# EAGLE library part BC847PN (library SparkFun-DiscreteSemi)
NPN/PNP transistor pair in SOT-363 package
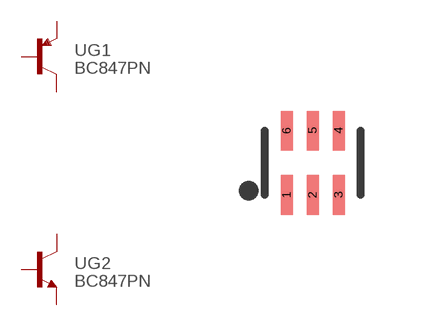
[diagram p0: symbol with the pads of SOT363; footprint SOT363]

Designator prefix -; gates G1=PNP G2=NPN

## BC847PN  [SOT363]
1  G1:E  pas
2  G1:B  pas
3  G2:C  pas
4  G2:E  pas
5  G2:B  pas
6  G1:C  pas

## Footprint SOT363 (pad centres in mm)
smd 0.3 x 0.99: 1 -0.65,-0.8; 2 0,-0.8; 3 0.65,-0.8; 4 0.65,0.81; 5 0,0.81; 6 -0.65,0.81

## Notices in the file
Licensing: CC v3.0 Share-Alike You are welcome to use this library for commercial purposes.
